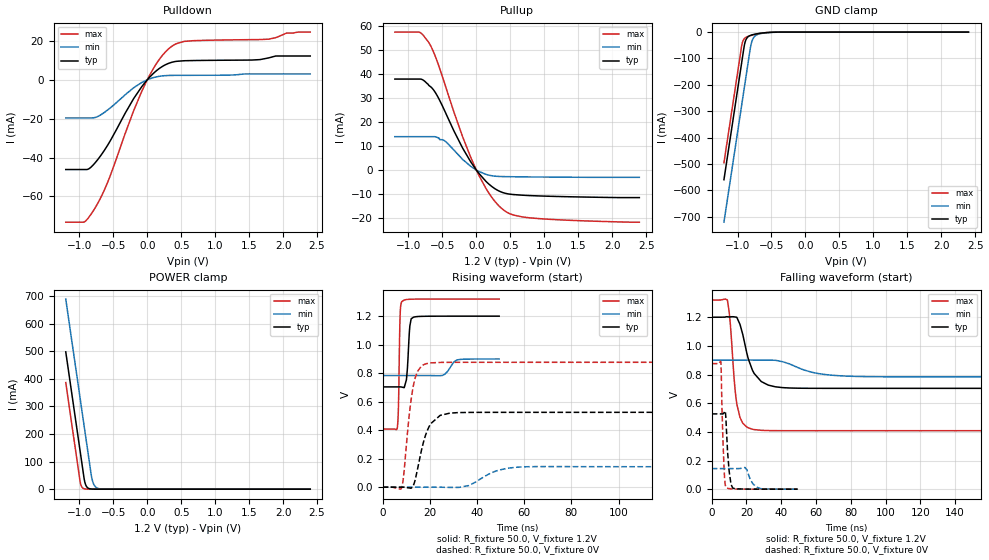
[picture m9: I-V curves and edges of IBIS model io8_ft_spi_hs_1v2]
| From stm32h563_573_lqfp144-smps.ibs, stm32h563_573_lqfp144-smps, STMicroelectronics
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[Model]   io8_ft_spi_hs_1v2
Model_type I/O
Polarity   Non-Inverting
Enable   Active-Low
| CAP_THRESHOLD on pad IOFT is "UDTCAPC" :
| Rising=20.0% of vddiom   Falling=80.0% of vddiom
| C_comp min and max val. don't necessarily correlate with the min and max pvt
| but are the smallest and greatest pad capacitance found.
| var   typ   min   max
C_comp   4.02960pF  3.92720pF  4.03450pF
|C_comp_pullup   2.45785pF  2.26900pF  2.18200pF
|C_comp_pulldown   1.57175pF  1.65820pF  1.85250pF
Vinl = 270.0mV
Vinh = 924.0mV
Vmeas = 600.0mV   | Reference voltage for timing measurements
Cref  = 50.0pF   | Timing specification test load capacitance value
Rref  = 100.0MOhm   | Timing specification test load resistance value
Vref  = 600.0mV   | Timing specification test load voltage
[Model Spec]
| TIME_THRESHOLD on pin ZIV11 is "CMOS" :
| Rising=40.0% of vdd   Falling=60.0% of vdd
Vinl 447.80000mV 344.80000mV 489.80000mV
Vinh 733.20000mV 535.20000mV 813.20000mV
| variable   typ   min   max
[Temperature Range] 25.0 125.0 -40.0
| variable   typ   min   max
[Voltage Range] 1.2V 900.0mV 1.32V
| variable   typ   min   max
[POWER Clamp Reference] 1.2V 900.0mV 1.32V
| variable   typ   min   max
[GND Clamp Reference] 0V 0V 0V
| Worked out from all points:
|   slope of the pulldown table from 0 to 0.18 V, typ, clamps not added: 30.6 ohm
|   slope of the pullup table from 0 to 0.18 V, typ, clamps not added: 31.3 ohm
|   GND clamp passes 1 mA (typ) near -0.52 V on its own axis
|   POWER clamp passes 1 mA (typ) near -0.84 V on its own axis
|   rising waveform, R_fixture 50.0, V_fixture 1.2V: 20-80 % time 1.03ns typ, 2.96ns min, 552ps max; typ from 0.704 V to 1.2 V
|   falling waveform, R_fixture 50.0, V_fixture 1.2V: 20-80 % time 7.35ns typ, 17.3ns min, 3.71ns max; typ from 1.2 V to 0.704 V
|   rising waveform, R_fixture 50.0, V_fixture 0V: 20-80 % time 5.04ns typ, 9.78ns min, 3.47ns max; typ from 0 V to 0.525 V
|   falling waveform, R_fixture 50.0, V_fixture 0V: 20-80 % time 1.81ns typ, 3.7ns min, 1.33ns max; typ from 0.525 V to 0 V
[POWER Clamp]
-1.2V     497.8mA    689.2mA    386.5mA
-990mV    140.8mA    332.2mA    29.53mA
-980mV    123.8mA    315.2mA    17.95mA
-960mV    89.81mA    281.2mA    6.634mA
-930mV    38.81mA    230.2mA    1.49mA
-900mV    12.07mA    179.2mA    334.8uA
-870mV    3.756mA    128.2mA    75.22uA
-820mV    536.4uA    44.98mA    6.246uA
-790mV    166.9uA    18.76mA    1.403uA
-750mV    35.18uA    5.846mA    191.9nA
-590mV    70.48nA    54.99uA    204.6pA
2.4V      0A         0A         0A
[GND Clamp]
-1.2V     -559.6mA   -720.6mA   -495.5mA
-940mV    -117.6mA   -278.6mA   -53.46mA
-930mV    -100.6mA   -261.6mA   -41.27mA
-900mV    -50.49mA   -210.6mA   -24.86mA
-880mV    -31.4mA    -176.6mA   -20.57mA
-850mV    -18.9mA    -125.6mA   -16.88mA
-810mV    -12.57mA   -58.3mA    -13.49mA
-780mV    -10.11mA   -29.57mA   -11.38mA
-740mV    -7.754mA   -14.31mA   -8.91mA
-640mV    -3.713mA   -4.821mA   -4.078mA
-390mV    -82.2uA    -288.6uA   -29.73uA
2.4V      3.859nA    727.3nA    172.3pA
| variable   typ   min   max
[Pullup Reference] 1.2V 900.0mV 1.32V
| variable   typ   min   max
[Pulldown Reference] 0V 0V 0V
[Pullup]
-1.2V     38.01mA    13.95mA    57.64mA
-840mV    38.01mA    13.95mA    57.59mA
-690mV    35.15mA    13.95mA    52.8mA
-600mV    32.21mA    13.85mA    47.19mA
-460mV    24.35mA    12.07mA    35.56mA
-200mV    9.064mA    4.397mA    13.74mA
0V        7.46pA     726pA      4.231pA
200mV     -6.245mA   -2.229mA   -10.29mA
400mV     -9.506mA   -2.731mA   -16.68mA
540mV     -10.23mA   -2.8mA     -18.76mA
790mV     -10.67mA   -2.88mA    -19.97mA
2.4V      -11.52mA   -3.045mA   -21.79mA
[Pulldown]
-1.2V     -46.17mA   -19.62mA   -73.27mA
-930mV    -46.17mA   -19.62mA   -73.17mA
-770mV    -42.8mA    -19.41mA   -66.04mA
-570mV    -32.88mA   -15.18mA   -51.58mA
-200mV    -9.658mA   -4.084mA   -15.89mA
-80mV     -3.488mA   -1.363mA   -5.887mA
130mV     4.529mA    1.469mA    8.049mA
340mV     8.782mA    2.251mA    16.66mA
540mV     9.805mA    2.305mA    19.74mA
1.79V     11.29mA    3.028mA    20.92mA
2.05V     12.25mA    3.028mA    24.04mA
2.4V      12.25mA    3.028mA    24.55mA
[Ramp]
dV/dt_r 315.16967mV/5.01402ns 86.13229mV/9.65856ns 525.78402mV/3.46307ns
dV/dt_f 297.79752mV/7.19054ns 69.92227mV/17.22184ns 547.13934mV/3.71175ns
R_load = 50.0
| Removed startup time: 0s 0s 0s  .
| Removed end time: 49.4ns.
[Rising Waveform]
R_fixture   = 50.0
V_fixture   = 1.2V
V_fixture_min = 900.0mV
V_fixture_max = 1.32V
0s        703.7mV    783.5mV    408.1mV
6.25ns    703.7mV    783.5mV    420.9mV
6.75ns    703.7mV    783.5mV    593.5mV
7.2ns     703.8mV    783.5mV    1.061V
7.4ns     703.8mV    783.5mV    1.198V
8.05ns    702.6mV    783.5mV    1.301V
10.1ns    754.6mV    783.5mV    1.317V
11.45ns   1.114V     783.5mV    1.318V
12.1ns    1.181V     783.5mV    1.319V
49.4ns    1.2V       899.8mV    1.32V
| Removed startup time: 0s 0s 0s  .
| Removed end time: 199.4ns.
[Falling Waveform]
R_fixture   = 50.0
V_fixture   = 1.2V
V_fixture_min = 900.0mV
V_fixture_max = 1.32V
0s        1.2V       900mV      1.32V
9ns       1.203V     900mV      1.319V
10.5ns    1.202V     900mV      1.179V
13ns      1.202V     900mV      754.2mV
14.5ns    1.198V     900mV      590.6mV
21.1ns    907.1mV    901.3mV    427.8mV
28.5ns    751mV      900.8mV    410.7mV
40.7ns    708.7mV    889.8mV    408.2mV
73.25ns   703.7mV    791.7mV    408.1mV
199.4ns   703.7mV    783.5mV    408.1mV
| Removed startup time: 0s 0s 0s  .
| Removed end time: 199.4ns.
[Rising Waveform]
R_fixture   = 50.0
V_fixture   = 0V
V_fixture_min = 0V
V_fixture_max = 0V
0s        166.5nV    850.9nV    114.4nV
8ns       95.39uV    1.152uV    -5.457mV
11.5ns    -5.742mV   1.11uV     538.1mV
13.1ns    14.87mV    959.9nV    717.3mV
14.8ns    126.6mV    713.3nV    812.2mV
18.8ns    392.2mV    2.081uV    867.7mV
24.4ns    503.9mV    -201.8uV   875.5mV
31.6ns    522.9mV    -1.69mV    876.1mV
57ns      525.2mV    140.3mV    876.3mV
199.4ns   525.3mV    143.6mV    876.3mV
| Removed startup time: 0s 0s 0s  .
| Removed end time: 49.4ns.
[Falling Waveform]
R_fixture   = 50.0
V_fixture   = 0V
V_fixture_min = 0V
V_fixture_max = 0V
0s        525.3mV    143.6mV    876.3mV
5.25ns    525.3mV    143.6mV    884.9mV
5.95ns    524.9mV    143.6mV    541.7mV
7.05ns    532.2mV    143.6mV    159.1mV
8.15ns    493.2mV    143.6mV    16.53mV
9.95ns    135.3mV    143.6mV    4.024mV
12.1ns    7.548mV    143.6mV    1.39mV
19.15ns   780.9uV    151mV      143.9uV
27.25ns   150.4uV    7.192mV    12.65uV
49.4ns    1.911uV    221.7uV    28.7nV
